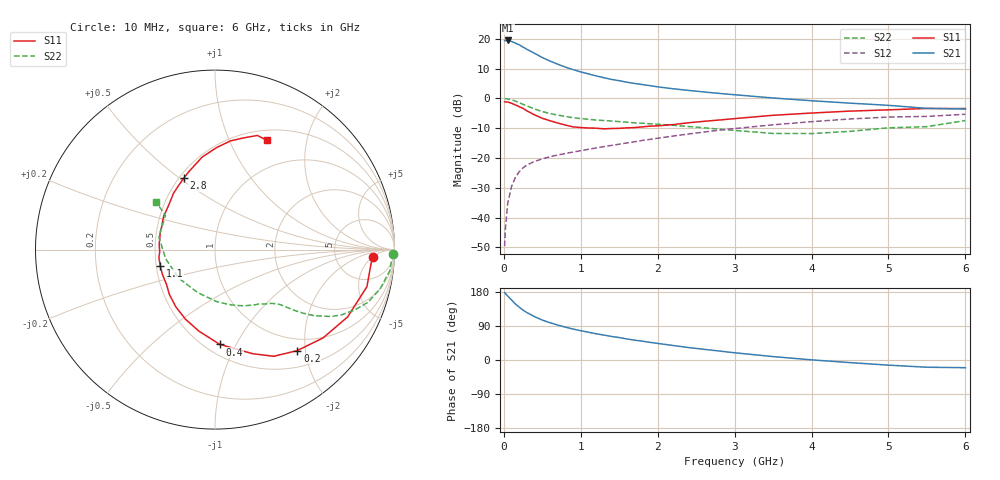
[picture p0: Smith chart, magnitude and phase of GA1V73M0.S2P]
! Infineon Technologies  Discrete & RF Semiconductors
! BF775
! Si NPN RF Bipolar Junction Transistor in SOT23
! VCE = 1.75 V  IC = 3 mA
! Common Emitter S-Parameters:  May  1996
# GHz  S  MA  R  50
!  f  S11  S21  S12  S22
! GHz  MAG  ANG  MAG  ANG  MAG  ANG  MAG  ANG
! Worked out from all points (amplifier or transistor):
!   36 points, 10 MHz to 6 GHz, reference 50 ohm
!   highest |S21| = 19.5 dB at 50 MHz (marker M1)
!   |S21| within 3 dB of that: start of sweep to 301.9 MHz
!   unconditionally stable (mu >= 1): 936.9 MHz to 4.327 GHz; 5.092 GHz to end of sweep
!   at 250 MHz: K = 0.37, MSG = 20.3 dB, |S12| = -23.3 dB
!   at 1.4 GHz: K = 1.15, MAG = 8.8 dB, |S12| = -15.8 dB
!   at 6 GHz: K = 1.01, MAG = 0.2 dB, |S12| = -5.3 dB
!   S11 on the Smith chart (normalised r, x): 10 MHz: 14, -5; 200 MHz: 0.78, -1.85; 400 MHz: 0.59, -0.86; 1.1 GHz: 0.53, -0.11; 2.8 GHz: 0.53, +0.52; 6 GHz: 0.62, +1.39
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0.01  0.8796 -2.8  9.366 178.0  0.0033 91.4  0.9937 -1.3
0.02  0.8728 -5.2  9.273 175.4  0.0064 87.8  0.9877 -2.7
0.05  0.8714 -13.7  9.4 168.9  0.0173 82.1  0.9807 -6.9
0.1  0.8288 -26.9  9.028 158.5  0.0331 75.1  0.9458 -13.4
0.15  0.7773 -39.3  8.484 147.9  0.047 68.6  0.9016 -19.0
0.2  0.7258 -50.8  7.958 139.4  0.0586 63.6  0.8463 -23.5
0.25  0.6789 -61.1  7.281 131.7  0.0682 58.9  0.7942 -27.2
0.3  0.617 -70.1  6.674 125.1  0.0762 56.0  0.7482 -29.9
0.4  0.5288 -87.1  5.715 114.4  0.0876 51.4  0.6638 -33.7
0.5  0.4633 -101.1  4.856 105.3  0.0965 49.2  0.6002 -36.0
0.6  0.4212 -113.0  4.236 98.4  0.105 47.7  0.5582 -37.4
0.7  0.3861 -124.5  3.759 92.2  0.112 47.3  0.5249 -38.4
0.9  0.3326 -144.3  3.045 81.7  0.1257 47.2  0.4741 -40.2
1.1  0.3185 -163.2  2.579 73.3  0.1399 47.7  0.4453 -42.5
1.4  0.3122 174.9  2.084 62.2  0.1624 48.0  0.4169 -46.5
1.6  0.3202 161.9  1.869 55.5  0.1787 48.1  0.3989 -49.5
2.2  0.3632 134.0  1.451 38.3  0.2331 46.6  0.3537 -62.2
2.8  0.4337 113.8  1.213 23.7  0.2925 42.2  0.3044 -80.3
3.5  0.5205 97.9  1.016 9.0  0.3602 34.6  0.258 -112.2
4.5  0.6118 81.9  0.832 -6.9  0.4512 21.9  0.2798 -169.5
5.5  0.6784 69.6  0.68 -19.1  0.4986 7.1  0.3357 145.3
6  0.6742 64.6  0.663 -20.3  0.5415 3.0  0.4248 141.0
